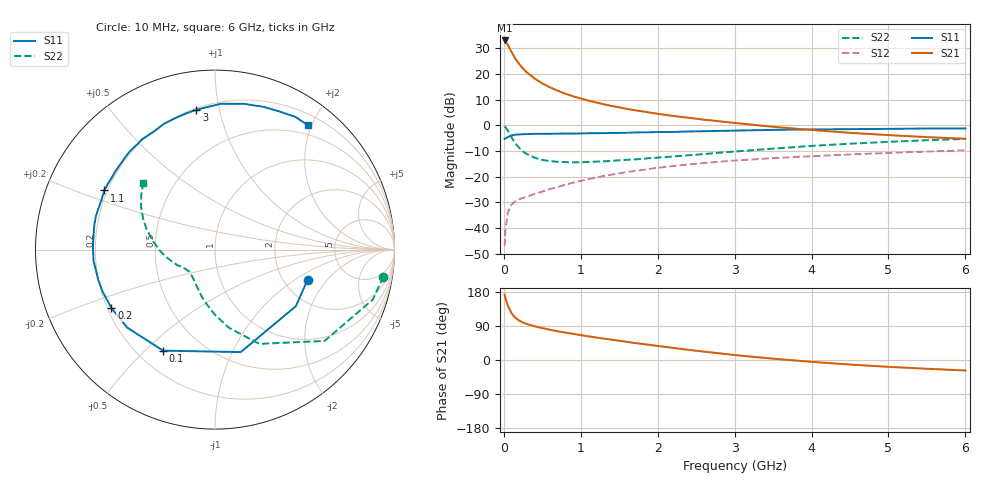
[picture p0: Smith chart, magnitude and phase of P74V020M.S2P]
! SIEMENS Small Signal Semiconductors
! BFP196
! Si NPN RF Bipolar Junction Transistor in SOT143
! VCE = 4 V  IC = 20 mA
! Common Emitter S-Parameters:  May  1996
# GHz  S  MA  R  50
!  f  S11  S21  S12  S22
! GHz  MAG  ANG  MAG  ANG  MAG  ANG  MAG  ANG
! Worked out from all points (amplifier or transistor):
!   36 points, 10 MHz to 6 GHz, reference 50 ohm
!   highest |S21| = 33.1 dB at 10 MHz (marker M1)
!   |S21| within 3 dB of that: start of sweep to 73.96 MHz
!   unconditionally stable (mu >= 1): 675 MHz to 3.417 GHz
!   at 250 MHz: K = 0.60, MSG = 25.2 dB, |S12| = -28.3 dB
!   at 1.4 GHz: K = 1.11, MAG = 11.4 dB, |S12| = -19.3 dB
!   at 6 GHz: K = 0.96, MSG = 2.3 dB, |S12| = -9.8 dB
!   S11 on the Smith chart (normalised r, x): 10 MHz: 2.68, -1.28; 100 MHz: 0.30, -0.57; 200 MHz: 0.22, -0.25; 1.1 GHz: 0.19, +0.24; 3 GHz: 0.21, +0.85; 6 GHz: 0.35, +1.94
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0.01  0.5426 -18.1  44.93 172.4  0.0044 82.6  0.9496 -9.1
0.02  0.5498 -35.0  43.21 163.7  0.009 75.8  0.9228 -17.5
0.05  0.5888 -75.9  37.24 144.4  0.0195 61.2  0.7949 -39.8
0.1  0.6329 -117.2  26.8 123.3  0.0285 47.6  0.5804 -64.8
0.15  0.6541 -138.3  19.84 111.3  0.0331 41.8  0.4423 -79.9
0.2  0.6627 -150.6  15.6 103.9  0.0362 40.4  0.361 -90.4
0.25  0.6683 -159.2  12.66 98.6  0.0384 40.9  0.3072 -98.7
0.3  0.6719 -165.3  10.7 94.9  0.0405 42.4  0.2751 -105.2
0.4  0.6797 -174.7  8.158 89.0  0.0459 44.8  0.2328 -115.1
0.5  0.68 179.0  6.54 84.2  0.0509 47.3  0.2108 -122.4
0.6  0.6813 173.2  5.473 79.8  0.0572 49.3  0.1998 -128.0
0.7  0.6867 168.1  4.713 75.7  0.0626 50.9  0.1939 -132.5
0.8  0.6892 164.1  4.123 72.3  0.0695 51.7  0.1915 -136.3
1.1  0.6993 151.9  3.019 62.5  0.0892 52.7  0.1931 -143.6
1.3  0.7015 144.8  2.563 56.4  0.1028 52.1  0.1984 -147.9
1.6  0.7154 135.1  2.084 47.9  0.1222 50.0  0.2124 -153.3
2.2  0.7399 117.7  1.519 32.0  0.1602 44.2  0.246 -163.4
3  0.7862 97.6  1.11 13.0  0.2054 34.3  0.3073 -178.9
3.5  0.8131 87.7  0.933 3.5  0.2282 28.2  0.3505 171.9
4.5  0.8403 71.1  0.712 -12.0  0.2702 16.9  0.4368 156.6
5.5  0.8645 58.7  0.587 -23.1  0.3068 6.1  0.5111 143.5
6  0.8649 53.3  0.545 -27.7  0.3241 0.3  0.5443 137.3
